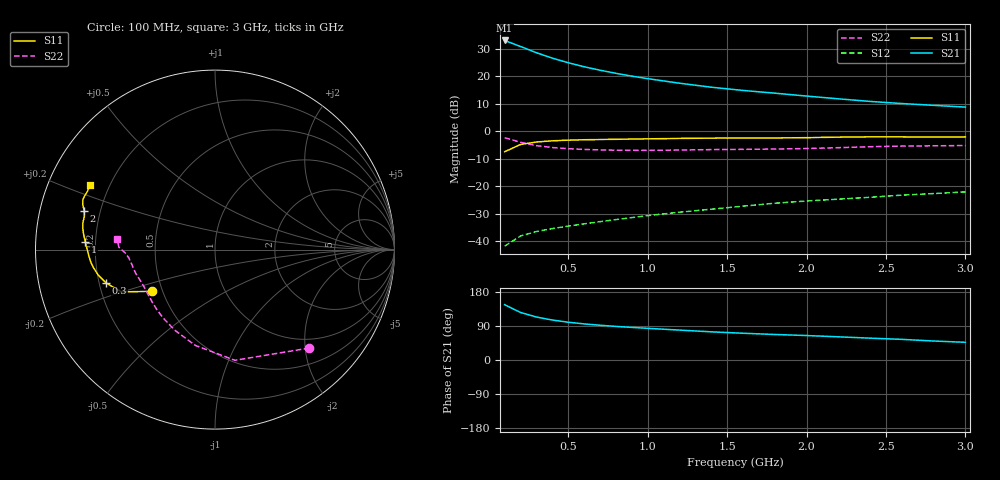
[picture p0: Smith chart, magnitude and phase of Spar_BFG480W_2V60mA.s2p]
! Filename: 260BFG480.001
! Title: BFG480W
! Bias: Vce=2V; Ic=60mA
! Company: NXP Semiconductors NL
! User: Quality&Reliability T&D
! Measure time: 10 Nov 1999 / 11:54:13
#  MHz  S  MA  R 50
! Freq  S11  S21  S12  S22  :
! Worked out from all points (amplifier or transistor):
!   20 points, 100 MHz to 3 GHz, reference 50 ohm
!   highest |S21| = 33.0 dB at 100 MHz (marker M1)
!   |S21| within 3 dB of that: start of sweep to 235.7 MHz
!   unconditionally stable (mu >= 1): 834.2 MHz to end of sweep
!   at 400 MHz: K = 0.72, MSG = 31.0 dB, |S12| = -35.5 dB
!   at 1.2 GHz: K = 1.07, MAG = 21.8 dB, |S12| = -29.5 dB
!   at 3 GHz: K = 1.10, MAG = 13.5 dB, |S12| = -22.1 dB
!   S11 on the Smith chart (normalised r, x): 100 MHz: 0.44, -0.25; 300 MHz: 0.23, -0.14; 1 GHz: 0.16, +0.03; 2 GHz: 0.14, +0.14; 3 GHz: 0.13, +0.24
100  0.4211 -146.5  44.76 145.9  0.008048 67.3  0.7594 -46.2
200  0.5706 -155.6  34.78 125.5  0.01233 56.3  0.6267 -79.8
300  0.6344 -162.9  26.8 113.4  0.01486 53.5  0.5449 -101.6
400  0.6664 -167.8  21.33 105.5  0.01681 54.1  0.5024 -116.3
500  0.6848 -171.6  17.6 99.7  0.01867 55.7  0.4789 -126.8
600  0.6969 -174.6  14.87 95.2  0.02049 57.4  0.4648 -134.5
700  0.7036 -177.1  12.87 91.7  0.02248 59.5  0.4554 -140.4
800  0.71 -179.4  11.29 88.6  0.02449 61.5  0.4495 -145.3
900  0.7176 178.5  10.04 86.0  0.02663 63.4  0.4467 -149.5
1000  0.7236 176.6  9.031 83.6  0.02896 64.7  0.4466 -153.1
1200  0.7367 173.4  7.459 78.9  0.03341 66.8  0.4528 -159.0
1400  0.746 170.9  6.31 74.3  0.03787 68.2  0.4613 -163.4
1600  0.7513 168.4  5.51 70.6  0.04307 69.4  0.4661 -166.9
1800  0.7509 165.7  4.913 67.3  0.0487 70.2  0.472 -170.5
2000  0.7604 163.4  4.349 64.6  0.05343 71.2  0.4823 -174.4
2200  0.7781 161.2  3.877 61.2  0.05771 71.3  0.4999 -177.8
2400  0.7866 159.4  3.474 57.6  0.06246 71.0  0.5203 -179.9
2600  0.7857 157.6  3.181 54.5  0.06842 70.5  0.5346 178.7
2800  0.781 155.3  2.947 50.1  0.07298 69.2  0.5403 176.8
3000  0.7853 152.6  2.738 46.7  0.07824 68.5  0.5467 173.9
